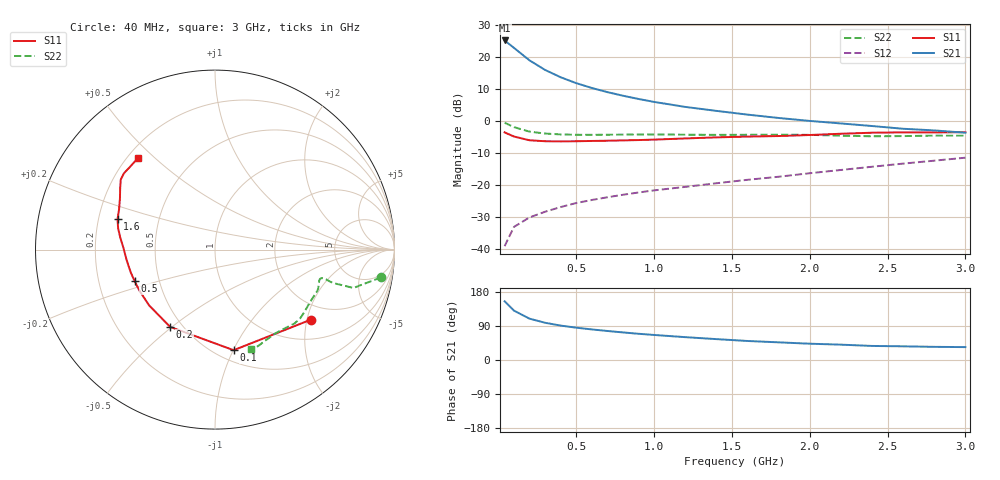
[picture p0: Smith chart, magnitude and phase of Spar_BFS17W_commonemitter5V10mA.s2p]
! Filename:  BFS17WC.S2P  Version:  4.0
! NXP part #: BFS17W  Date: Jun 1994
! Bias condition: Vce=5V, Ic=10mA
#  MHz  S  MA  R  50
! Freq  S11  S21  S12  S22  !GUM [dB]
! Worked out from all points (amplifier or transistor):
!   21 points, 40 MHz to 3 GHz, reference 50 ohm
!   highest |S21| = 25.2 dB at 40 MHz (marker M1)
!   |S21| within 3 dB of that: start of sweep to 117.5 MHz
!   unconditionally stable (mu >= 1): 398 MHz to 2.28 GHz
!   at 300 MHz: K = 0.89, MSG = 22.2 dB, |S12| = -28.4 dB
!   at 1 GHz: K = 1.20, MAG = 11.1 dB, |S12| = -21.7 dB
!   at 3 GHz: K = 0.96, MSG = 3.9 dB, |S12| = -11.5 dB
!   S11 on the Smith chart (normalised r, x): 40 MHz: 1.52, -2.12; 100 MHz: 0.60, -1.00; 200 MHz: 0.43, -0.49; 500 MHz: 0.36, -0.16; 1.6 GHz: 0.28, +0.14; 3 GHz: 0.24, +0.44
40  0.662 -36.1  18.12 154.9  0.011 73.3  0.938 -9.5
100  0.57 -79.5  13.88 130.3  0.022 59.3  0.8 -15.5
200  0.498 -120.1  8.849 109.1  0.031 54.8  0.68 -15.8
300  0.481 -139.8  6.272 98.2  0.038 56.2  0.635 -14.9
400  0.479 -151.3  4.817 90.8  0.045 58.8  0.615 -14.9
500  0.481 -158.7  3.895 85.3  0.052 61.2  0.607 -15.6
600  0.486 -164.5  3.276 80.7  0.058 63.7  0.606 -16.7
700  0.49 -169.2  2.821 76.6  0.064 65.1  0.608 -17.9
800  0.496 -173.4  2.478 72.8  0.07 67.0  0.611 -19.2
900  0.502 -177.3  2.204 69.2  0.076 68.4  0.614 -20.4
1000  0.51 179.0  1.983 66.1  0.082 69.9  0.615 -21.7
1200  0.532 172.8  1.656 60.3  0.093 73.1  0.609 -25.1
1400  0.553 167.5  1.436 55.1  0.106 76.4  0.605 -29.5
1600  0.569 162.6  1.255 50.2  0.12 79.4  0.607 -34.5
1800  0.58 157.1  1.112 46.6  0.134 82.6  0.61 -38.7
2000  0.602 151.6  1 43.0  0.152 85.2  0.605 -42.8
2200  0.63 147.0  0.913 40.5  0.171 87.2  0.588 -47.8
2400  0.654 143.4  0.832 37.1  0.192 88.7  0.575 -54.3
2600  0.662 140.0  0.754 36.1  0.215 89.1  0.579 -60.9
2800  0.661 135.4  0.71 34.7  0.239 89.5  0.589 -66.1
3000  0.667 129.9  0.654 34.0  0.266 89.4  0.587 -70.3
